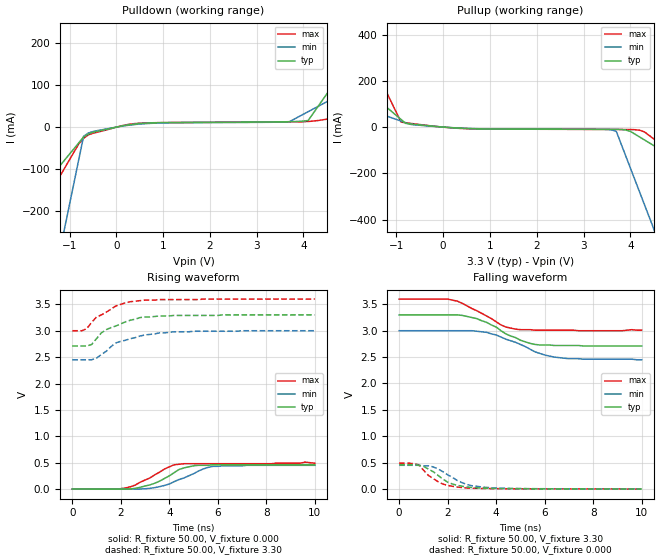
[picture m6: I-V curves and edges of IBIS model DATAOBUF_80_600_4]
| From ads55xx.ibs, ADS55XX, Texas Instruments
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|   Model DATAOBUF_80_600_4
[Model]   DATAOBUF_80_600_4
Model_type   Output
Polarity   Non-Inverting
Vmeas =   1.65V
C_comp   3.00pF   3.00pF   3.00pF
[Temperature Range]   50.00   0.10k   -20.00
[Voltage Range]   3.30V   3.00V   3.60V
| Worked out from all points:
|   slope of the pulldown table from 0 to 0.495 V, typ, clamps not added: 58.8 ohm
|   slope of the pullup table from 0 to 0.495 V, typ, clamps not added: 81.2 ohm
|   rising waveform, R_fixture 50.00, V_fixture 0.000: 20-80 % time 1.11ns typ, 1.34ns min, 1.18ns max; typ from 0 V to 0.46 V
|   rising waveform, R_fixture 50.00, V_fixture 3.30: 20-80 % time 1.32ns typ, 1.5ns min, 1.13ns max; typ from 2.71 V to 3.3 V
|   falling waveform, R_fixture 50.00, V_fixture 3.30: 20-80 % time 1.51ns typ, 1.72ns min, 1.39ns max; typ from 3.3 V to 2.71 V
|   falling waveform, R_fixture 50.00, V_fixture 0.000: 20-80 % time 965ps typ, 1.08ns min, 845ps max; typ from 0.46 V to 0.001 V
[Pulldown]
| voltage   I(typ)   I(min)   I(max)
-3.3V     -375.1mA   -1.424A    -515.9mA
-2.3V     -239.9mA   -884.9mA   -325.3mA
-1.9V     -185.8mA   -669.2mA   -249.1mA
-1.5V     -131.7mA   -453.5mA   -172.8mA
-1V       -64.1mA    -183.8mA   -77.52mA
-700mV    -23.54mA   -22.03mA   -26.56mA
-500mV    -12.41mA   -10.44mA   -14.63mA
500mV     8.47mA     7.27mA     9.4mA
3.7V      12.9mA     12.99mA    12.43mA
4.1V      15.75mA    36.75mA    13.47mA
5.5V      237.8mA    119.9mA    35.77mA
6.6V      412.2mA    185.2mA    54.3mA
[Pullup]
| voltage   I(typ)   I(min)   I(max)
-3.3V     442mA      197.8mA    1.021A
-3.1V     408mA      183.5mA    937.3mA
-1.9V     203.6mA    97.69mA    438mA
-900mV    33.33mA    26.19mA    21.87mA
-800mV    16.3mA     19.04mA    18.86mA
400mV     -4.88mA    -4.43mA    -5.85mA
3.6V      -9.51mA    -11.92mA   -9.95mA
3.7V      -9.63mA    -18.5mA    -9.99mA
4V        -18.21mA   -176.7mA   -10.36mA
4.2V      -42.85mA   -282.1mA   -13.47mA
4.5V      -79.81mA   -440.3mA   -50.82mA
6.6V      -338.5mA   -1.547A    -370mA
[Ramp]
| variable   typ   min   max
dV/dt_r   0.28/1.19n   0.27/1.35n   0.29/1.14n
dV/dt_f   0.35/1.51n   0.33/1.68n   0.36/1.39n
R_load = 50.00
[Rising Waveform]
R_fixture = 50.00
V_fixture = 0.000
V_fixture_min = 0.000
V_fixture_max = 0.000
| time   V(typ)   V(min)   V(max)
0s        15.67nV    19.34nV    32.63nV
1.8ns     -1.9mV     -1.13mV    110uV
2.6ns     12.73mV    -2.05mV    75.41mV
3.2ns     78.74mV    13.12mV    210mV
3.8ns     200mV      68.27mV    380mV
4.2ns     310mV      140mV      460mV
4.6ns     400mV      210mV      480mV
5.4ns     450mV      380mV      480mV
5.8ns     460mV      430mV      480mV
10ns      460mV      450mV      490mV
[Rising Waveform]
R_fixture = 50.00
V_fixture = 3.30
V_fixture_min = 3.00
V_fixture_max = 3.60
| time   V(typ)   V(min)   V(max)
0s        2.71V      2.45V      3V
600ps     2.71V      2.45V      3.04V
800ps     2.74V      2.45V      3.16V
1ns       2.85V      2.48V      3.26V
1.4ns     3.02V      2.61V      3.35V
1.8ns     3.09V      2.77V      3.47V
2.4ns     3.2V       2.85V      3.55V
2.8ns     3.25V      2.9V       3.57V
4.2ns     3.29V      2.98V      3.59V
10ns      3.3V       3V         3.6V
[Falling Waveform]
R_fixture = 50.00
V_fixture = 3.30
V_fixture_min = 3.00
V_fixture_max = 3.60
| time   V(typ)   V(min)   V(max)
0s        3.3V       3V         3.6V
2ns       3.3V       3V         3.6V
2.4ns     3.3V       3V         3.56V
3.2ns     3.23V      2.99V      3.38V
3.6ns     3.16V      2.97V      3.28V
4.2ns     3V         2.88V      3.11V
4.8ns     2.87V      2.78V      3.03V
5.6ns     2.74V      2.6V       3.01V
6.4ns     2.72V      2.5V       3.01V
10ns      2.71V      2.45V      3.01V
[Falling Waveform]
R_fixture = 50.00
V_fixture = 0.000
V_fixture_min = 0.000
V_fixture_max = 0.000
| time   V(typ)   V(min)   V(max)
0s        460mV      450mV      490mV
800ps     450mV      450mV      460mV
1.2ns     380mV      440mV      260mV
1.4ns     330mV      420mV      200mV
1.8ns     190mV      330mV      94.68mV
2ns       130mV      270mV      68.89mV
2.6ns     53.01mV    120mV      27.74mV
3ns       28.8mV     62.49mV    14.8mV
4.2ns     8.98mV     16.07mV    5.72mV
10ns      1.46mV     1.8mV      1.24mV
